(* Logix 5000 Rung export; software revision 16.03 *)

TYPE MNETCRETHERNET :   // Stores the MVI56E-MNETCR IP settings
STRUCT
   IP : INT[4];   // Module IP address
   Netmask : INT[4];   // Net mask used by the Module
   Gateway : INT[4];   // Gateway used by the module
END_STRUCT
END_TYPE

TYPE MNETCRETHERNETTYPE :   // Allows read/write Ethernet settings between the module and processor
STRUCT
   Read : BOOL;   // Enable Ethernet configuration transfer from module to processor
   Write : BOOL;   // Enable Ethernet configuration transfer from processor to module
   Config : MNETCRETHERNET;   // Module ethernet configurations ip, netmask and gateway
END_STRUCT
END_TYPE

TYPE MNETCRDATETIME :   // Stores the date and time value
STRUCT
   Year : DINT;   // Displays module current year
   Month : DINT;   // Displays Module current month
   Day : DINT;   // Displays Module current day
   Hour : DINT;   // Displays Module current hour
   Minute : DINT;   // Displays Module current minute
   Seconds : DINT;   // Displays Module current second
END_STRUCT
END_TYPE

TYPE MNETCRCLOCKTYPE :   // Allows read/write of clock value between the module and processor
STRUCT
   Read : BOOL;   // Reads current time from the module
   Write : BOOL;   // Writes current time from the module
   Config : MNETCRDATETIME;   // Date and time configuration read or written between the module and processor
END_STRUCT
END_TYPE

ADD_ON_INSTRUCTION AOI56EMNETCR_OPTIONAL   (* revision 1.0, vendor ProSoft Technology Inc. *)
// MVI56E-MNETCR Optional Add-On Ethernet/Clock
// Revision note:
// Release
VAR_IN_OUT
   MVI56MNETCREthernet : MNETCRETHERNETTYPE; {required}   // MVI56E-MNET Rev2 Ethernet Settings
   MVI56MNETCRClock : MNETCRCLOCKTYPE; {required}   // MVI56E-MNET Rev2 Clock Settings
   ReadEthernetMSG : MESSAGE; {required}   // Read Ethernet Settings Message
   WriteEthernetMSG : MESSAGE; {required}   // Write Ethernet Settings Message
   ReadClockMSG : MESSAGE; {required}   // Read Clock Settings Message
   WriteClockMSG : MESSAGE; {required}   // Write Clock Settings Message
END_VAR

ROUTINE Logic   (* ladder *)
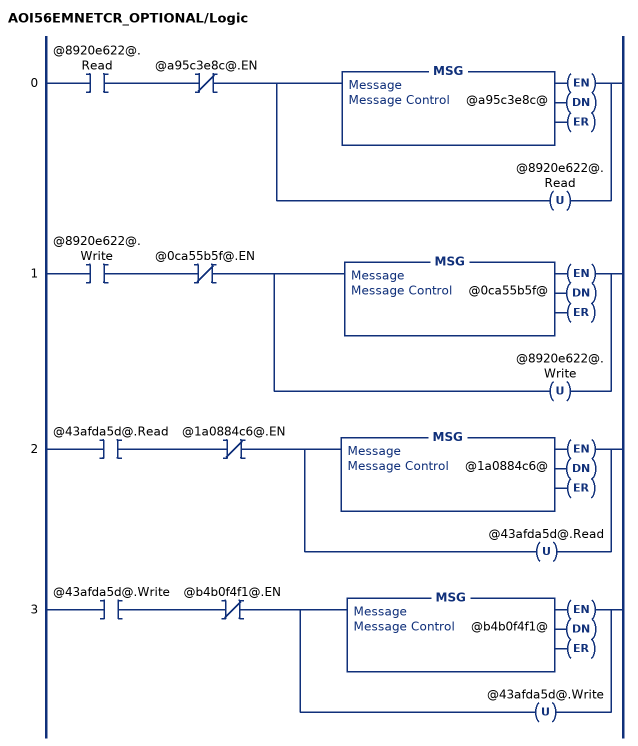
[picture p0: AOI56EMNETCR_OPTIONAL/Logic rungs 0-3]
   0: XIC(@8920e622@.Read)XIO(@a95c3e8c@.EN)[MSG(@a95c3e8c@) ,OTU(@8920e622@.Read) ];
   1: XIC(@8920e622@.Write)XIO(@0ca55b5f@.EN)[MSG(@0ca55b5f@) ,OTU(@8920e622@.Write) ];
   2: XIC(@43afda5d@.Read)XIO(@1a0884c6@.EN)[MSG(@1a0884c6@) ,OTU(@43afda5d@.Read) ];
   3: XIC(@43afda5d@.Write)XIO(@b4b0f4f1@.EN)[MSG(@b4b0f4f1@) ,OTU(@43afda5d@.Write) ];
END_ROUTINE
END_ADD_ON_INSTRUCTION

VAR_GLOBAL   (* controller tags *)
   READCLOCKMSG : MESSAGE;
        MessageParameters(MessageType := CIP Generic, ConnectedFlag := 2, ConnectionPath := MNETCR, ServiceCode := 16#000e, ObjectType := 16#0004, TargetObject := 8, AttributeNumber := 16#0020, DestinationTag := MVI56EMNETCRCLOCK.Config)
   READETHERNETMSG : MESSAGE;
        MessageParameters(MessageType := CIP Generic, ConnectedFlag := 2, ConnectionPath := MNETCR, ServiceCode := 16#000e, ObjectType := 16#0004, TargetObject := 8, DestinationTag := MVI56EMNETCRETHERNET.Config)
   MVI56EMNETCRCLOCK : MNETCRCLOCKTYPE;
   WRITEETHERNETMSG : MESSAGE;
        MessageParameters(MessageType := CIP Generic, RequestedLength := 24, ConnectedFlag := 2, ConnectionPath := MNETCR, ServiceCode := 16#0010, ObjectType := 16#0004, TargetObject := 8, LocalElement := MVI56EMNETCRETHERNET.Config)
   WRITECLOCKMSG : MESSAGE;
        MessageParameters(MessageType := CIP Generic, RequestedLength := 24, ConnectedFlag := 2, ConnectionPath := MNETCR, ServiceCode := 16#0010, ObjectType := 16#0004, TargetObject := 8, AttributeNumber := 16#0020, LocalElement := MVI56EMNETCRCLOCK.Config)
   MVI56EMNETCRETHERNET : MNETCRETHERNETTYPE;
   AOI56EMNETCR_OPTIONAL : AOI56EMNETCR_OPTIONAL;
END_VAR

PROGRAM MainProgram

ROUTINE MainRoutine   (* ladder *)
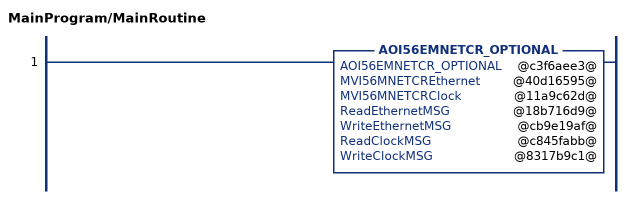
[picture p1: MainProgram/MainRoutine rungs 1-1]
   1: AOI56EMNETCR_OPTIONAL(@c3f6aee3@,@40d16595@,@11a9c62d@,@18b716d9@,@cb9e19af@,@c845fabb@,@8317b9c1@);
END_ROUTINE
END_PROGRAM
